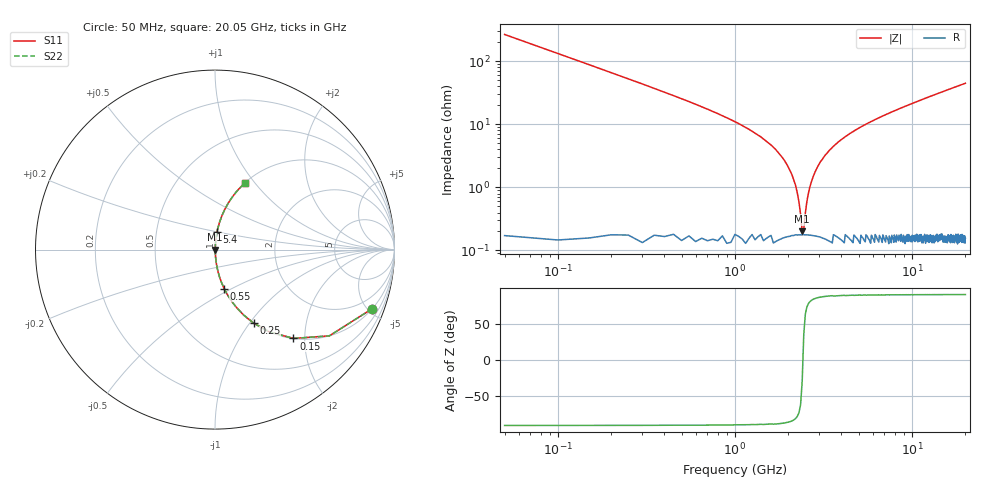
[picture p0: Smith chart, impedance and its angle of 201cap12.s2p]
! AVX Thin Film Operation		Date: May 2007
! Description: Accu-P® Series, Thin Film, SMD, RF Capacitor
! Part Number: 0201ZK120FBS
! 50 MHz  -  20.05 GHz
! Serial Measurements
# MHZ S MA R 50
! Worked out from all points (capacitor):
!   401 points, 50 MHz to 20.05 GHz, reference 50 ohm
!   read as one part in series: C = 12 pF near 150 MHz
!   lowest |Z| = 203 mohm at 2.4 GHz (marker M1)
!   series resonance near 2.422 GHz, so ESL is about 360 pH
!   S11 on the Smith chart (normalised r, x): 50 MHz: 1.01, -5.30; 150 MHz: 1.00, -1.76; 250 MHz: 1.00, -1.05; 550 MHz: 1.00, -0.46; 5.4 GHz: 1.00, +0.20; 20.05 GHz: 1.00, +0.89
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50  0.935 -20.7  0.353 69.3  0.353 69.3  0.935 -20.7
150  0.66 -48.6  0.75 41.3  0.75 41.3  0.66 -48.6
250  0.464 -62.2  0.884 27.7  0.884 27.7  0.464 -62.2
350  0.347 -69.4  0.936 20.3  0.936 20.3  0.347 -69.4
550  0.223 -76.7  0.973 12.9  0.973 12.9  0.223 -76.7
1050  0.102 -83.3  0.993 5.8  0.993 5.8  0.102 -83.3
1900  0.027 -85.2  0.998 1.5  0.998 1.5  0.027 -85.2
2150  0.013 -82.5  0.998 0.7  0.998 0.7  0.013 -82.5
2350  0.003624 -64.5  0.998 0.2  0.998 0.2  0.003624 -64.5
2400  0.001829 -32.1  0.998 0.1  0.998 0.1  0.001829 -32.1
2500  0.003819 65.9  0.998 -0.2  0.998 -0.2  0.003819 65.9
2650  0.009998 80.5  0.998 -0.6  0.998 -0.6  0.009998 80.5
2800  0.016 83.5  0.998 -0.9  0.998 -0.9  0.016 83.5
3050  0.026 85.1  0.998 -1.5  0.998 -1.5  0.026 85.1
3400  0.038 85.5  0.998 -2.2  0.998 -2.2  0.038 85.5
4250  0.065 84.9  0.996 -3.7  0.996 -3.7  0.065 84.9
5400  0.097 83.5  0.994 -5.6  0.994 -5.6  0.097 83.5
6750  0.132 81.8  0.99 -7.6  0.99 -7.6  0.132 81.8
10050  0.209 77.5  0.976 -12.1  0.976 -12.1  0.209 77.5
13400  0.281 73.4  0.958 -16.3  0.958 -16.3  0.281 73.4
16750  0.347 69.4  0.936 -20.3  0.936 -20.3  0.347 69.4
20050  0.407 65.8  0.912 -24.0  0.912 -24.0  0.407 65.8
